(* Logix 5000 AddOnInstructionDefinition export AMCI_SV160E2_Preset_on_Enable; software revision 20.03 *)

ADD_ON_INSTRUCTION AMCI_SV160E2_Preset_on_Enable   (* revision 1.0, vendor AMCI, ExecuteEnableInFalse *)
// Revision note:
// 8/2019 Version 0 Initial release of SV160E2 Add On Instructions.
// 3/17/20 Version 1 replaced the generic EDS file with a more complete V1.6 EDS file.
VAR_IN_OUT
   AMCI_SV160E2_output_data : _000A:SV160E2_9125ACD4:O:0; {required}
END_VAR
VAR_OUTPUT
   EN : BOOL; {access Read Only, visible}
END_VAR
VAR
   command_data_block : INT[10];
        [0]   // Command Word 0
        [1]   // Command Word 1
        [3]   // Lower Target Position
        [5]   // Lower Programmed Speed
END_VAR

ROUTINE EnableInFalse   (* ladder *)
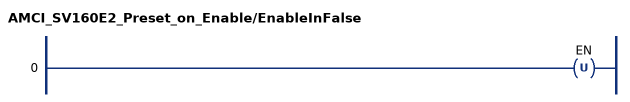
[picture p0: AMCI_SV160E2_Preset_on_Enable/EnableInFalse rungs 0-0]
   0: OTU(EN);
END_ROUTINE

ROUTINE Logic   (* ladder *)
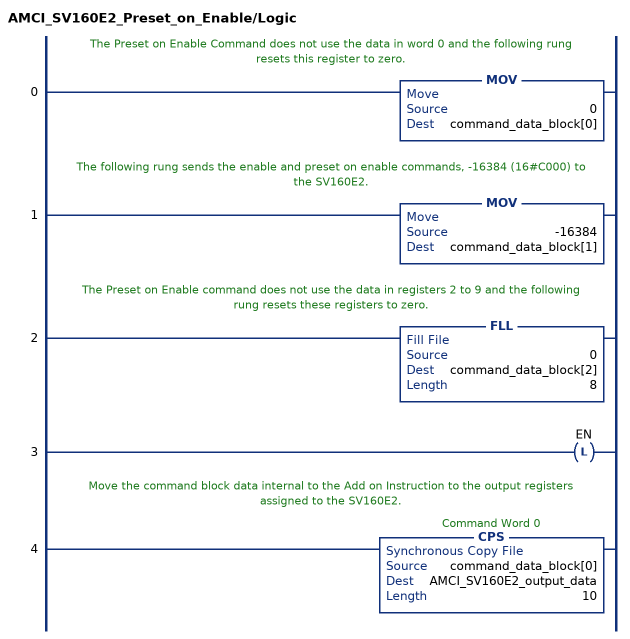
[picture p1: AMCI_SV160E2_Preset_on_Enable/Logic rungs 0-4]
   // The Preset on Enable Command does not use the data in word 0 and the following rung resets this register to zero.
   0: MOV(0,command_data_block[0]);
   // The following rung sends the enable and preset on enable commands, -16384 (16#C000) to the SV160E2.
   1: MOV(-16384,command_data_block[1]);
   // The Preset on Enable command does not use the data in registers 2 to 9 and the following rung resets these registers to zero.
   2: FLL(0,command_data_block[2],8);
   3: OTL(EN);
   // Move the command block data internal to the Add on Instruction to the output registers assigned to the SV160E2.
   4: CPS(command_data_block[0],AMCI_SV160E2_output_data,10);
END_ROUTINE
END_ADD_ON_INSTRUCTION
